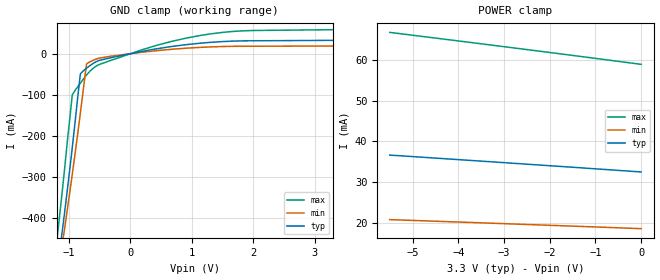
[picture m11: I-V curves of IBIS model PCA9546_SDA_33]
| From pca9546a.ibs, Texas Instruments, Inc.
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[Model]   PCA9546_SDA_33
Model_type  Terminator
| variable   typ   min   max
C_comp   6.35pF   5.03pF   8.37pF
| C_tri-state   6.35pF   5.03pF   8.37pF
[Temperature Range]   40   100   -40
| Ambient temperature   25   85   -40
[Voltage range]   3.3   3   3.6
[GND Clamp]
| PCA9546_SDA_33
|   Voltage   I(typ)   I(min)   I(max)
-5.5V     -4.144A    -3.967A    -4.348A
-1.195V   -535.9mA   -554.2mA   -456.3mA
-1.15V    -484.4mA   -509.6mA   -396mA
-1.105V   -431.5mA   -464.2mA   -333.4mA
-1.065V   -383.3mA   -423.2mA   -275.6mA
-945mV    -230.6mA   -295.8mA   -102.3mA
-810mV    -48.94mA   -142.7mA   -71.5mA
-715mV    -35.88mA   -29.18mA   -52.74mA
-685mV    -32.41mA   -22.29mA   -47.45mA
185mV     5.474mA    3.396mA    9.246mA
1.14V     25.6mA     15.38mA    44.44mA
3.3V      32.49mA    18.68mA    58.51mA
[POWER Clamp]
| PCA9546_SDA_33
|   Voltage   I(typ)   I(min)   I(max)
-5.5V     36.64mA    20.77mA    66.81mA
-2.49V    34.4mA     19.58mA    62.58mA
-1.105V   33.35mA    19.01mA    60.58mA
-95.1fV   32.49mA    18.55mA    58.96mA
